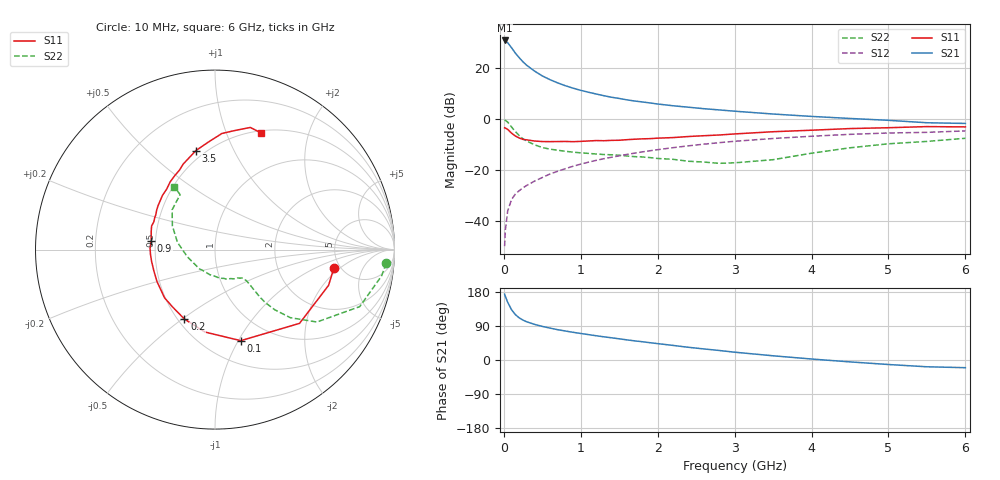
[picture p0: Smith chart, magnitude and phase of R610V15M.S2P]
! SIEMENS Small Signal Semiconductors
! BFR193
! Si NPN RF Bipolar Junction Transistor in SOT23
! VCE = 10 V  IC = 15 mA
! Common Emitter S-Parameters:  May  1996
# GHz  S  MA  R  50
!  f  S11  S21  S12  S22
! GHz  MAG  ANG  MAG  ANG  MAG  ANG  MAG  ANG
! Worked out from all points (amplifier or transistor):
!   36 points, 10 MHz to 6 GHz, reference 50 ohm
!   highest |S21| = 30.8 dB at 10 MHz (marker M1)
!   |S21| within 3 dB of that: start of sweep to 103.6 MHz
!   unconditionally stable (mu >= 1): 676.9 MHz to 2.112 GHz
!   at 250 MHz: K = 0.74, MSG = 24.7 dB, |S12| = -27.0 dB
!   at 1.4 GHz: K = 1.04, MAG = 10.6 dB, |S12| = -15.0 dB
!   at 6 GHz: K = 0.94, MSG = 1.5 dB, |S12| = -4.7 dB
!   S11 on the Smith chart (normalised r, x): 10 MHz: 4.44, -1.63; 100 MHz: 0.73, -1.02; 200 MHz: 0.54, -0.51; 900 MHz: 0.47, +0.05; 3.5 GHz: 0.45, +0.72; 6 GHz: 0.53, +1.33
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0.01  0.6704 -8.7  34.65 173.7  0.0032 77.5  0.9571 -4.6
0.02  0.6634 -17.5  33.91 167.8  0.0067 76.9  0.9389 -9.1
0.05  0.6251 -41.1  31.36 152.3  0.0157 70.9  0.8666 -21.5
0.1  0.5273 -74.2  24.97 132.7  0.0263 62.7  0.6965 -35.4
0.15  0.4628 -96.9  19.54 119.7  0.0337 59.3  0.5658 -42.1
0.2  0.423 -113.7  15.89 111.2  0.0392 59.1  0.4721 -45.2
0.25  0.3974 -126.6  13.16 105.1  0.0448 59.8  0.4075 -46.5
0.3  0.3888 -136.3  11.21 100.6  0.05 60.6  0.3664 -46.6
0.4  0.369 -151.2  8.667 94.0  0.0605 62.6  0.3111 -45.9
0.5  0.3605 -161.0  6.994 88.6  0.0711 64.4  0.2755 -45.2
0.6  0.3593 -169.4  5.894 84.2  0.0834 65.1  0.2559 -44.8
0.7  0.3606 -176.0  5.099 80.0  0.0941 65.7  0.2436 -44.8
0.9  0.3585 172.3  4.017 73.1  0.1182 65.5  0.2232 -45.8
1.1  0.3703 163.6  3.343 67.0  0.1421 64.6  0.2113 -48.8
1.3  0.3743 155.6  2.859 61.2  0.1662 62.9  0.2008 -52.1
1.6  0.3925 145.9  2.369 53.1  0.2017 60.2  0.1876 -59.7
2.2  0.4314 128.6  1.815 38.5  0.2735 53.5  0.1616 -80.6
3  0.5084 110.4  1.42 20.6  0.365 42.3  0.138 -129.0
3.5  0.562 100.9  1.25 11.1  0.4138 34.9  0.159 -165.3
4.5  0.6481 86.6  1.023 -5.0  0.4992 20.8  0.2721 150.8
5.5  0.7083 73.9  0.843 -17.9  0.5462 6.3  0.363 122.4
6  0.6989 68.4  0.817 -20.3  0.5834 2.1  0.4179 123.0
